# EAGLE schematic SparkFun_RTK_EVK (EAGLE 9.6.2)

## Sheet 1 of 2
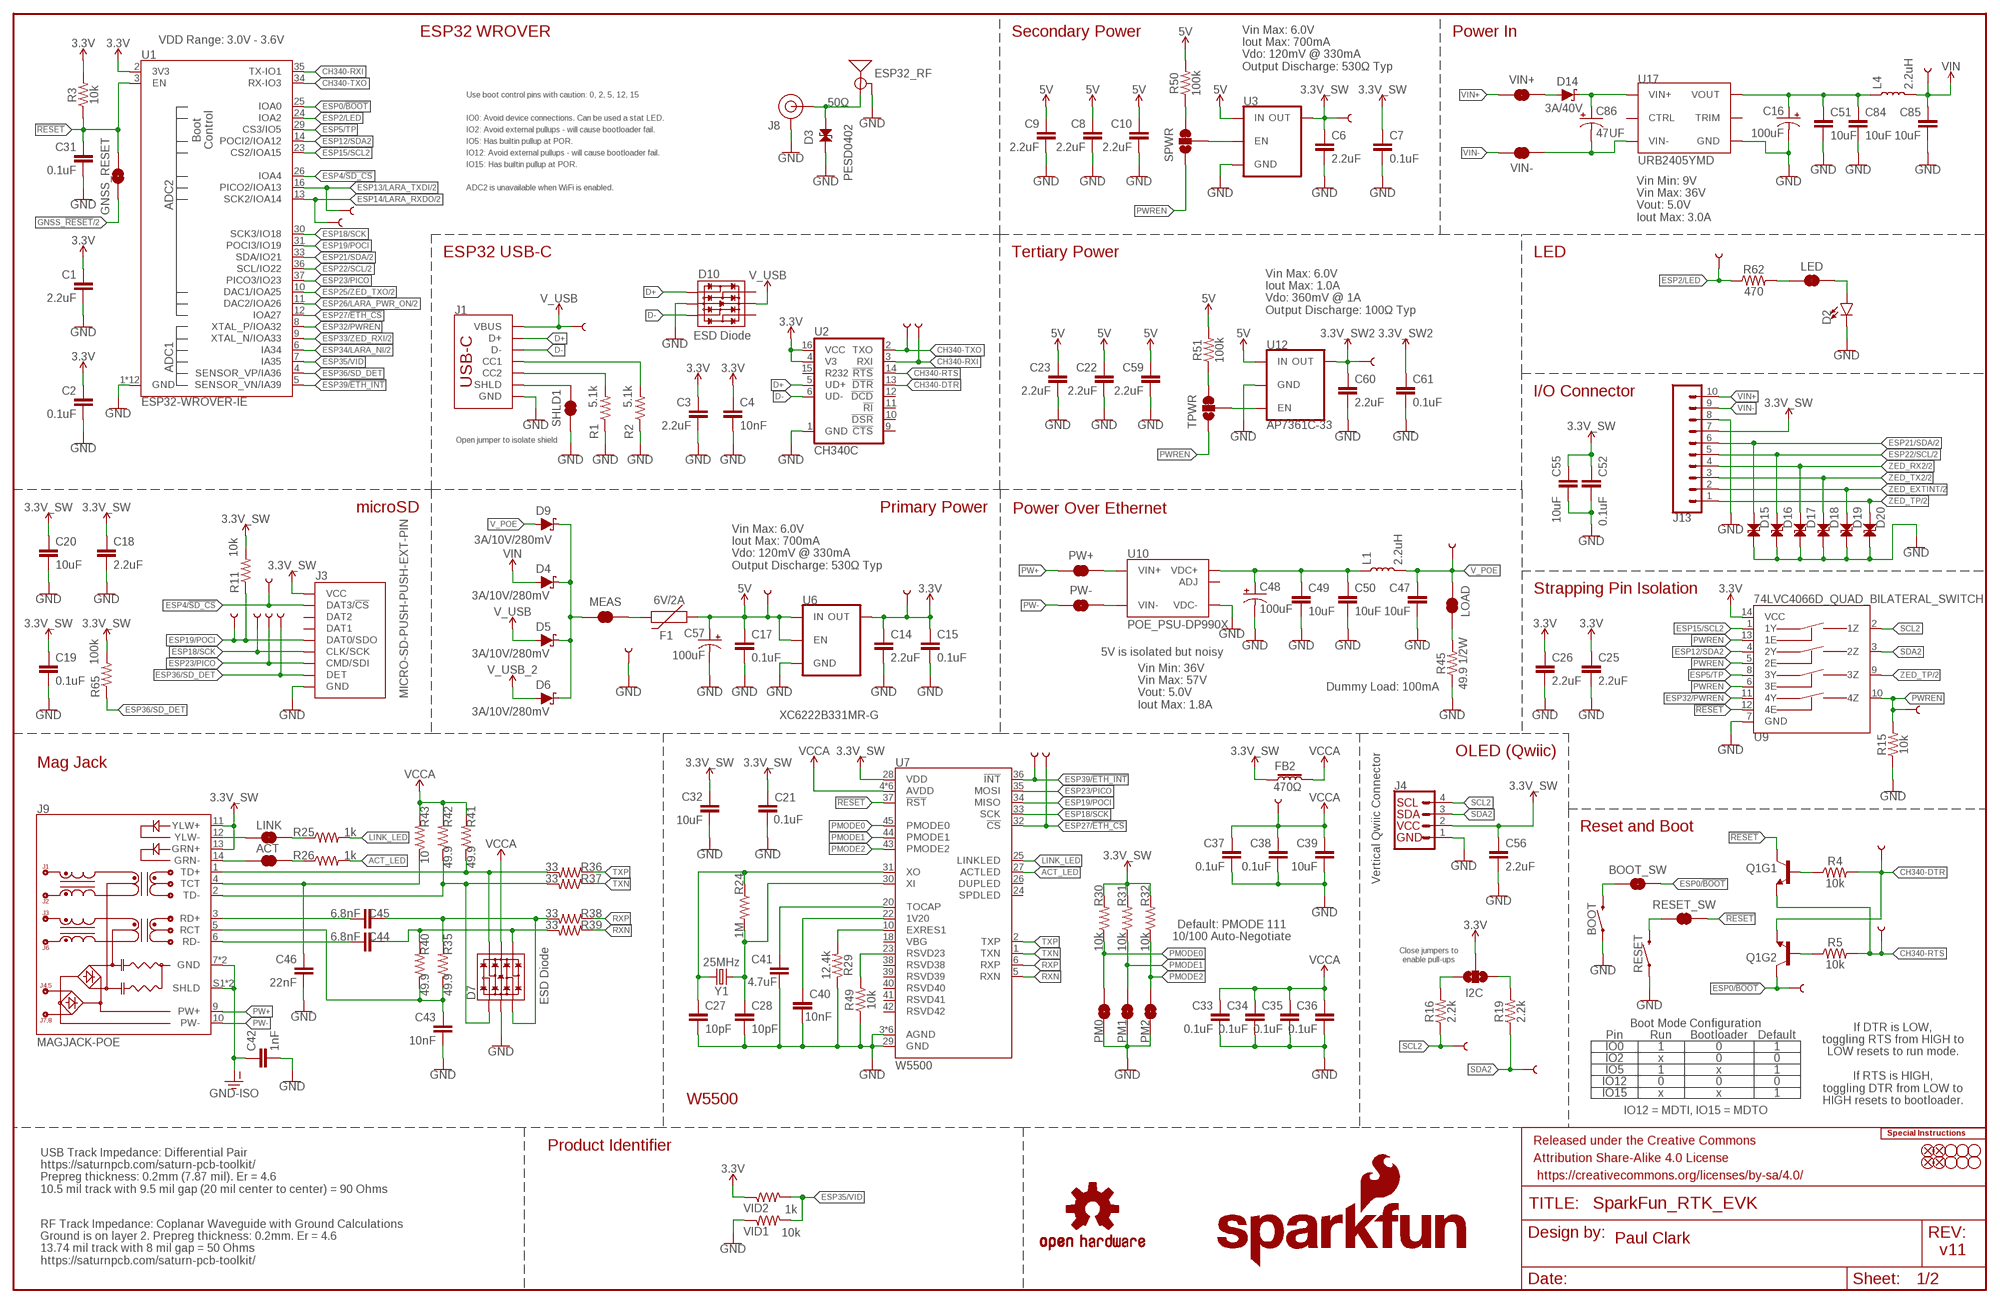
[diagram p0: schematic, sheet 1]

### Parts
3V3  TEST-POINTPOGO_PTH  [1X01_NO_SILK]
3V3_SW  TEST-POINTPOGO_PTH  [1X01_NO_SILK]
3V3_SW2  TEST-POINTPOGO_PTH  [1X01_NO_SILK]
5V  TEST-POINTPOGO_PTH  [1X01_NO_SILK]
ACT  JUMPER-SMT_2_NC_TRACE_SILK  [SMT-JUMPER_2_NC_TRACE_SILK]
BOOT  MOMENTARY-SWITCH-SPST-PTH-RIGHT-ANGLE-8-020  [TACTILE_SWITCH_PTH_RA_8-020]
BOOT_SW  JUMPER-SMT_2_NC_TRACE_SILK  [SMT-JUMPER_2_NC_TRACE_SILK]
C1  2.2uF  2.2UF-0603-10V-20%  [0603]
C2  0.1uF  0.1UF-0603-25V-5%  [0603]
C3  2.2uF  2.2UF-0603-10V-20%  [0603]
C4  10nF  10NF-0603-50V-10%  [0603]
C6  2.2uF  2.2UF-0603-10V-20%  [0603]
C7  0.1uF  0.1UF-0603-25V-5%  [0603]
C8  2.2uF  2.2UF-0603-10V-20%  [0603]
C9  2.2uF  2.2UF-0603-10V-20%  [0603]
C10  2.2uF  2.2UF-0603-10V-20%  [0603]
C14  2.2uF  2.2UF-0603-10V-20%  [0603]
C15  0.1uF  0.1UF-0603-25V-5%  [0603]
C16  100uF  100UF-POLAR-25V-20%(ELEC)  [PANASONIC_D]
C17  0.1uF  0.1UF-0603-25V-5%  [0603]
C18  2.2uF  2.2UF-0603-10V-20%  [0603]
C19  0.1uF  0.1UF-0603-25V-5%  [0603]
C20  10uF  10UF-0603-6.3V-20%  [0603]
C21  0.1uF  0.1UF-0603-25V-5%  [0603]
C22  2.2uF  2.2UF-0603-10V-20%  [0603]
C23  2.2uF  2.2UF-0603-10V-20%  [0603]
C25  2.2uF  2.2UF-0603-10V-20%  [0603]
C26  2.2uF  2.2UF-0603-10V-20%  [0603]
C27  10pF  10PF-0603-50V-5%  [0603]
C28  10pF  10PF-0603-50V-5%  [0603]
C31  0.1uF  0.1UF-0603-25V-5%  [0603]
C32  10uF  10UF-0603-6.3V-20%  [0603]
C33  0.1uF  0.1UF-0603-25V-5%  [0603]
C34  0.1uF  0.1UF-0603-25V-5%  [0603]
C35  0.1uF  0.1UF-0603-25V-5%  [0603]
C36  0.1uF  0.1UF-0603-25V-5%  [0603]
C37  0.1uF  0.1UF-0603-25V-5%  [0603]
C38  0.1uF  0.1UF-0603-25V-5%  [0603]
C39  10uF  10UF-0603-6.3V-20%  [0603]
C40  10nF  10NF-0603-50V-10%  [0603]
C41  4.7uF  4.7UF-0603-6.3V-(10%)  [0603]
C42  1nF  1.0NF/1000PF-1206-2KV-10%  [1206]
C43  10nF  10NF-0603-50V-10%  [0603]
C44  6.8nF  6.8NF/6800PF-0603-50V-5%  [0603]
C45  6.8nF  6.8NF/6800PF-0603-50V-5%  [0603]
C46  22nF  22NF/22,000PF-0603-50V-10%  [0603]
C47  10uF  10UF-0805-25V-10%  [0805]
C48  100uF  100UF-POLAR-25V-20%(ELEC)  [PANASONIC_D]
C49  10uF  10UF-0805-25V-10%  [0805]
C50  10uF  10UF-0805-25V-10%  [0805]
C51  10uF  10UF-0805-25V-10%  [0805]
C52  0.1uF  0.1UF-0603-25V-5%  [0603]
C55  10uF  10UF-0603-6.3V-20%  [0603]
C56  2.2uF  2.2UF-0603-10V-20%  [0603]
C57  100uF  100UF-POLAR-25V-20%(ELEC)  [PANASONIC_D]
C59  2.2uF  2.2UF-0603-10V-20%  [0603]
C60  2.2uF  2.2UF-0603-10V-20%  [0603]
C61  0.1uF  0.1UF-0603-25V-5%  [0603]
C84  10uF  10UF-0805-25V-10%  [0805]
C85  10uF  10UF-0805-25V-10%  [0805]
C86  47UF  47UF-POLAR-PANASONIC_D-50V-20%  [PANASONIC_D]
D2  LED-RIGHT-ANGLE-PTH-GREEN  [CBI-RIGHT-ANGLE-PTH]
D3  PESD0402  PESD0402-0402  [0402]
D4  3A/10V/280mV  DIODE-SCHOTTKY-BAT60A  [SOD-323]
D5  3A/10V/280mV  DIODE-SCHOTTKY-BAT60A  [SOD-323]
D6  3A/10V/280mV  DIODE-SCHOTTKY-BAT60A  [SOD-323]
D7  ESD Diode  TVS_DIODE_ARRAY_DT1042-04SO-7  [SOT-23-6]
D9  3A/10V/280mV  DIODE-SCHOTTKY-BAT60A  [SOD-323]
D10  ESD Diode  TVS_DIODE_ARRAY_DT1042-04SO-7  [SOT-23-6]
D14  3A/40V  DIODE-SCHOTTKY-B340A  [SMA-DIODE]
D15  PESD0402-0402  [0402]
D16  PESD0402-0402  [0402]
D17  PESD0402-0402  [0402]
D18  PESD0402-0402  [0402]
D19  PESD0402-0402  [0402]
D20  PESD0402-0402  [0402]
DET  TEST-POINTPOGO_PTH  [1X01_NO_SILK]
DTR  TEST-POINTPOGO_PTH  [1X01_NO_SILK]
ESP32_RF  ANTENNA-SMA-GROUNDEDEDGE_RPSMA  [RP-SMA-EDGE]
ETH_CS  TEST-POINTPOGO_PTH  [1X01_NO_SILK]
ETH_INT  TEST-POINTPOGO_PTH  [1X01_NO_SILK]
F1  6V/2A  PPTC_6V2A  [1210]
FB2  470Ω  FERRITE_BEAD-0603-470Ω-100MHZ-1A-200MILIΩ  [0603]
FD1  FIDUCIAL1X2  [FIDUCIAL-1X2]
FD2  FIDUCIAL1X2  [FIDUCIAL-1X2]
FD3  FIDUCIAL1X2  [FIDUCIAL-1X2]
FD4  FIDUCIAL1X2  [FIDUCIAL-1X2]
FRAME1  FRAME-LEDGER  [CREATIVE_COMMONS]
GND  TEST-POINTPOGO_PTH  [1X01_NO_SILK]
GNSS_RESET  JUMPER-COMBO_2_NO  [COMBO-JUMPER_2_NO]
H1  STAND-OFFTIGHT  [STAND-OFF-TIGHT]
H2  STAND-OFFTIGHT  [STAND-OFF-TIGHT]
H3  STAND-OFFTIGHT  [STAND-OFF-TIGHT]
H4  STAND-OFFTIGHT  [STAND-OFF-TIGHT]
H5  STAND-OFFTIGHT  [STAND-OFF-TIGHT]
H6  STAND-OFFTIGHT  [STAND-OFF-TIGHT]
I2C  JUMPER-SMT_3_NO_SILK  [SMT-JUMPER_3_NO_SILK]
J1  USB_C_4-LAYER_PADS  [USB-C-16P_4LAYER-PADS]
J3  MICRO-SD-PUSH-PUSH-EXT-PIN  [MICROSD-EXTERNALPIN]
J4  Vertical Qwiic Connector  QWIIC_CONNECTOR  [JST04_1MM_VERT]
J8  U.FL2PIN-REDUCED-FOOTPRINT  [U.FL_REDUCED_FOOTPRINT]
J9  MAGJACK-POE  [MAGJACK-SYM_LED]
J13  CONN_10_3.5MM_RA_HEADER  [1X10_SCREW_TERMINAL_3.5MM]
L1  2.2uH  INDUCTOR-0805_WIDE-2.2UH  [0805-WIDE]
L4  2.2uH  INDUCTOR-0805_WIDE-2.2UH  [0805-WIDE]
LED  JUMPER-SMT_2_NC_TRACE_SILK  [SMT-JUMPER_2_NC_TRACE_SILK]
LINK  JUMPER-SMT_2_NC_TRACE_SILK  [SMT-JUMPER_2_NC_TRACE_SILK]
LOAD  JUMPER-SMT_2_NC_TRACE_SILK  [SMT-JUMPER_2_NC_TRACE_SILK]
LOGO1  SPECIAL_INSTRUCTIONS-ORDERING  [ORDERING_INSTRUCTIONS]
LOGO4  OSHW-LOGOS  [OSHW-LOGO-S]
LOGO5  SFE_LOGO_NAME.2_INCH  [SFE_LOGO_NAME_.2]
LOGO6  SFE_LOGO_FLAME.2_INCH  [SFE_LOGO_FLAME_.2]
MEAS  JUMPER-COMBO_2_NC_TRACE  [COMBO-JUMPER_2_NC_TRACE]
PICO  TEST-POINTPOGO_PTH  [1X01_NO_SILK]
PM0  JUMPER-SMT_2_NO_SILK  [SMT-JUMPER_2_NO_SILK]
PM1  JUMPER-SMT_2_NO_SILK  [SMT-JUMPER_2_NO_SILK]
PM2  JUMPER-SMT_2_NO_SILK  [SMT-JUMPER_2_NO_SILK]
POCI  TEST-POINTPOGO_PTH  [1X01_NO_SILK]
PW+  JUMPER-COMBO_2_NC_TRACE  [COMBO-JUMPER_2_NC_TRACE]
PW-  JUMPER-COMBO_2_NC_TRACE  [COMBO-JUMPER_2_NC_TRACE]
PWREN  TEST-POINTPOGO_PTH  [1X01_NO_SILK]
Q1  TRANS_NPN_DUAL-MBT3904DW1T1  [SC70-6]
R1  5.1k  5.1KOHM5.1KOHM-0603-1/10W-1%  [0603]
R2  5.1k  5.1KOHM5.1KOHM-0603-1/10W-1%  [0603]
R3  10k  10KOHM-0603-1/10W-1%  [0603]
R4  10k  10KOHM-0603-1/10W-1%  [0603]
R5  10k  10KOHM-0603-1/10W-1%  [0603]
R11  10k  10KOHM-0603-1/10W-1%  [0603]
R15  10k  10KOHM-0603-1/10W-1%  [0603]
R16  2.2k  2.2KOHM-0603-1/10W-1%  [0603]
R19  2.2k  2.2KOHM-0603-1/10W-1%  [0603]
R24  1M  1MOHM-0603-1/4W-5%  [0603]
R25  1k  1KOHM-0603-1/10W-1%  [0603]
R26  1k  1KOHM-0603-1/10W-1%  [0603]
R29  12.4k  12.4KOHM-0603-1/10W-1%  [0603]
R30  10k  10KOHM-0603-1/10W-1%  [0603]
R31  10k  10KOHM-0603-1/10W-1%  [0603]
R32  10k  10KOHM-0603-1/10W-1%  [0603]
R35  49.9  49.9OHM-0603-1/10W-1%  [0603]
R36  33  33OHM-0603-1/10W-1%  [0603]
R37  33  33OHM-0603-1/10W-1%  [0603]
R38  33  33OHM-0603-1/10W-1%  [0603]
R39  33  33OHM-0603-1/10W-1%  [0603]
R40  49.9  49.9OHM-0603-1/10W-1%  [0603]
R41  49.9  49.9OHM-0603-1/10W-1%  [0603]
R42  49.9  49.9OHM-0603-1/10W-1%  [0603]
R43  10  10OHM-0603-1/10W-1%  [0603]
R45  49.9 1/2W  49.9OHM-1206-1/2W-1%  [1206]
R49  10k  10KOHM-0603-1/10W-1%  [0603]
R50  100k  100KOHM-0603-1/10W-1%  [0603]
R51  100k  100KOHM-0603-1/10W-1%  [0603]
R62  470  470OHM-0603-1/10W-1%  [0603]
R65  100k  100KOHM-0603-1/10W-1%  [0603]
RESET  MOMENTARY-SWITCH-SPST-PTH-RIGHT-ANGLE-8-020  [TACTILE_SWITCH_PTH_RA_8-020]
RESET_SW  JUMPER-SMT_2_NC_TRACE_SILK  [SMT-JUMPER_2_NC_TRACE_SILK]
RTS  TEST-POINTPOGO_PTH  [1X01_NO_SILK]
RX  TEST-POINTPOGO_PTH  [1X01_NO_SILK]
RXD  TEST-POINTPOGO_PTH  [1X01_NO_SILK]
SCK  TEST-POINTPOGO_PTH  [1X01_NO_SILK]
SCL2  TEST-POINTPOGO_PTH  [1X01_NO_SILK]
SD_CS  TEST-POINTPOGO_PTH  [1X01_NO_SILK]
SDA2  TEST-POINTPOGO_PTH  [1X01_NO_SILK]
SHLD1  JUMPER-SMT_2_NC_TRACE_SILK  [SMT-JUMPER_2_NC_TRACE_SILK]
SPWR  JUMPER-SMT_3_1-NC_TRACE_SILK  [SMT-JUMPER_3_1-NC_TRACE_SILK]
TP_BOOT  TEST-POINTPOGO_PTH  [1X01_NO_SILK]
TP_LED  TEST-POINTPOGO_PTH  [1X01_NO_SILK]
TPWR  JUMPER-SMT_3_1-NC_TRACE_SILK  [SMT-JUMPER_3_1-NC_TRACE_SILK]
TX  TEST-POINTPOGO_PTH  [1X01_NO_SILK]
TXD  TEST-POINTPOGO_PTH  [1X01_NO_SILK]
U1  ESP32-WROVER-IE  ESP32-WROVER-E/IE_IE-N16R8  [ESP32-WROVER-E/IE]
U2  CH340C  [SO016]
U3  XC6222B331MR-G  [SOT23-5]
U6  XC6222B331MR-G  [SOT23-5]
U7  W5500  [LQFP-48]
U9  74LVC4066D_QUAD_BILATERAL_SWITCH  [SO14]
U10  POE_PSU-DP990X  [DP990X]
U12  AP7361C-33  AP7361C-33FGEUDFN-8  [UDFN-8]
U17  URB2405YMD  URB_YMD-15WR3__URB2405YMD-15WR3  [URB_YMD-15WR3]
VCCA  TEST-POINTPOGO_PTH  [1X01_NO_SILK]
VID1  10k  10KOHM-0603-1/10W-1%  [0603]
VID2  1k  1KOHM-0603-1/10W-1%  [0603]
VIN  TEST-POINTPOGO_PTH  [1X01_NO_SILK]
VIN+  JUMPER-COMBO_2_NC_TRACE  [COMBO-JUMPER_2_NC_TRACE]
VIN-  JUMPER-COMBO_2_NC_TRACE  [COMBO-JUMPER_2_NC_TRACE]
VPOE  TEST-POINTPOGO_PTH  [1X01_NO_SILK]
VUSB  TEST-POINTPOGO_PTH  [1X01_NO_SILK]
Y1  25MHz  CRYSTAL-25MHZ-SMD-2.0X1.6MM  [CRYSTAL-SMD-2.0X1.6MM]

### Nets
3.3V: 3V3.1 C1.1 C2.1 C3.1 C4.1 C14.1 C15.1 C25.1 C26.1 I2C.2 R3.2 U1.2(3V3) U2.4(V3) U2.16(VCC) U6.5(OUT) U9.14(VCC) VID2.1
3.3V_SW: 3V3_SW.1 C6.1 C7.1 C18.1 C19.1 C20.1 C21.1 C32.1 C52.1 C55.1 C56.1 FB2.1 J3.4(VCC) J4.2 J9.11(YLW+) J9.13(GRN+) J13.7 R11.2 R30.2 R31.2 R32.2 R65.2 U3.5(OUT) U7.28(VDD) ; also sheet 2
3.3V_SW2: 3V3_SW2.1 C60.1 C61.1 U12.1(OUT) ; also sheet 2
5V: 5V.1 C8.1 C9.1 C10.1 C17.1 C22.1 C23.1 C57.+ C59.1 F1.1 R50.2 R51.2 U3.1(IN) U6.1(IN) U6.3(EN) U12.8(IN) ; also sheet 2
5V_RAW: C48.+ C49.1 C50.1 L1.1 U10.1(VDC+) U10.2(VDC+)
5V_RAW1: C16.+ C51.1 C84.1 L4.1 U17.4(VOUT)
!RESET!: C31.1 GNSS_RESET.2 GNSS_RESET.4 Q1.3(C) R3.1 RESET_SW.1 U1.3(EN) U7.37(!RST!) U9.12(4E)
ACT: ACT.1 J9.14(GRN-)
ACT_LED: R26.2 U7.27(ACTLED)
CH340-DTR: DTR.1 Q1.1(E) R4.2 U2.13(!DTR)
CH340-RTS: Q1.4(E) R5.2 RTS.1 U2.14(!RTS)
CH340-RXI: TX.1 U1.35(TX-IO1) U2.3(RXI)
CH340-TXO: RX.1 U1.34(RX-IO3) U2.2(TXO)
D+: D10.1(IO1) J1.A6(D+) J1.B6(D+) U2.5(UD+)
D-: D10.3(IO2) J1.A7(D-) J1.B7(D-) U2.6(UD-)
ESP0/!BOOT!: BOOT_SW.1 Q1.6(C) TP_BOOT.1 U1.25(IOA0)
ESP2/LED: R62.1 TP_LED.1 U1.24(IOA2)
ESP4/!SD_CS!: J3.2(DAT3/!CS!) SD_CS.1 U1.26(IOA4)
ESP5/TP: U1.29(CS3/IO5) U9.8(3Y)
ESP12/SDA2: U1.14(POCI2/IOA12) U9.4(2Y)
ESP13/LARA_TXDI: TXD.1 U1.16(PICO2/IOA13) ; also sheet 2
ESP14/LARA_RXDO: RXD.1 U1.13(SCK2/IOA14) ; also sheet 2
ESP15/SCL2: U1.23(CS2/IOA15) U9.1(1Y)
ESP18/SCK: J3.5(CLK/SCK) SCK.1 U1.30(SCK3/IO18) U7.33(SCK)
ESP19/POCI: J3.7(DAT0/SDO) POCI.1 R11.1 U1.31(POCI3/IO19) U7.34(MISO)
ESP21/SDA: D15.1 J13.6 U1.33(SDA/IO21) ; also sheet 2
ESP22/SCL: D16.1 J13.5 U1.36(SCL/IO22) ; also sheet 2
ESP23/PICO: J3.3(CMD/SDI) PICO.1 U1.37(PICO3/IO23) U7.35(MOSI)
ESP25/ZED_TXO: U1.10(DAC1/IOA25) ; also sheet 2
ESP26/LARA_PWR_ON: U1.11(DAC2/IOA26) ; also sheet 2
ESP27/!ETH_CS!: ETH_CS.1 U1.12(IOA27) U7.32(!CS!)
ESP32/PWREN: U1.8(XTAL_P/IOA32) U9.11(4Y)
ESP33/ZED_RXI: U1.9(XTAL_N/IOA33) ; also sheet 2
ESP34/LARA_NI: U1.6(IA34) ; also sheet 2
ESP35/VID: U1.7(IA35) VID1.2 VID2.2
ESP36/SD_DET: DET.1 J3.9(DET) R65.1 U1.4(SENSOR_VP/IA36)
ESP39/!ETH_INT!: ETH_INT.1 U1.5(SENSOR_VN/IA39) U7.36(!INT!)
GND: BOOT.1 C1.2 C2.2 C3.2 C4.2 C6.2 C7.2 C8.2 C9.2 C10.2 C14.2 C15.2 C16.- C17.2 C18.2 C19.2 C20.2 C21.2 C22.2 C23.2 C25.2 C26.2 C27.2 C28.2 C31.2 C32.2 C33.2 C34.2 C35.2 C36.2 C37.2 C38.2 C39.2 C40.2 C41.2 C42.2 C43.2 C46.2 C47.2 C48.- C49.2 C50.2 C51.2 C52.2 C55.2 C56.2 C57.- C59.2 C60.2 C61.2 C84.2 C85.2 D2.C D3.2 D7.2(VSS) D10.2(VSS) D15.2 D16.2 D17.2 D18.2 D19.2 D20.2 ESP32_RF.GND@0(GND) ESP32_RF.GND@1(GND) ESP32_RF.GND@2(GND) ESP32_RF.GND@3(GND) GND.1 J1.GND J1.GND2(GND) J3.6(GND) J3.10(GND) J3.11(GND) J3.12(GND) J3.13(GND) J4.1 J8.1(GND) J8.2(GND) J13.8 PM0.1 PM1.1 PM2.1 R1.1 R2.1 R15.1 R29.1 R45.1 R49.1 RESET.1 SHLD1.1 U1.1(GND) U1.15(GND) U1.38(GND) U1.GND U1.GNDT1(GND) U1.GNDT2(GND) U1.GNDT3(GND) U1.GNDT4(GND) U1.GNDT5(GND) U1.GNDT6(GND) U1.GNDT7(GND) U1.GNDT8(GND) U2.1(GND) U3.2(GND) U6.2(GND) U7.3(AGND) U7.9(AGND) U7.14(AGND) U7.16(AGND) U7.19(AGND) U7.29(GND) U7.48(AGND) U9.7(GND) U10.3(VDC-) U12.4(GND) U12.EP(GND) U17.6(GND) VID1.1 ; also sheet 2
GND-ISO: C42.1 J9.7(GND) J9.8(GND) J9.S1(SHLD) J9.S2(SHLD)
GNSS_!RESET!: GNSS_RESET.1 GNSS_RESET.3 ; also sheet 2
LINK: J9.12(YLW-) LINK.1
LINK_LED: R25.2 U7.25(LINKLED)
MEAS: D4.C D5.C D6.C D9.C MEAS.2 MEAS.4
N$1: J1.B5(CC2) R1.2
N$2: J1.A5(CC1) R2.2
N$4: Q1.2(B) R5.1
N$5: Q1.5(B) R4.1
N$7: LED.2 R62.2
N$10: F1.2 MEAS.1 MEAS.3
N$12: ACT.2 R26.1
N$13: D3.1 ESP32_RF.SIG(SIGNAL) J8.FEED(SIGNAL)
N$14: I2C.3 R16.2
N$15: I2C.1 R19.2
N$19: C27.1 R24.1 U7.31(XO) Y1.1
N$20: C28.1 R24.2 U7.30(XI) Y1.3
N$21: LINK.2 R25.1
N$22: R50.1 SPWR.3
N$23: R29.2 U7.10(EXRES1)
N$24: C40.1 U7.22(1V20)
N$25: C41.1 U7.20(TOCAP)
N$26: SPWR.2 U3.3(EN)
N$27: LOAD.1 R45.2
N$28: RESET.2 RESET_SW.2
N$29: BOOT.2 BOOT_SW.2
N$30: R49.2 U7.23(RSVD23)
N$31: R51.1 TPWR.3
N$39: TPWR.2 U12.5(EN)
N$45: D2.A LED.1
PMODE0: PM0.2 R30.1 U7.45(PMODE0)
PMODE1: PM1.2 R31.1 U7.44(PMODE1)
PMODE2: PM2.2 R32.1 U7.43(PMODE2)
PW1+: PW+.1 PW+.3 U10.5(VIN+) U10.6(VIN+)
PW1-: PW-.1 PW-.3 U10.7(VIN-) U10.8(VIN-)
PW+: J9.9(PW+) PW+.2 PW+.4
PW-: J9.10(PW-) PW-.2 PW-.4
PWREN: PWREN.1 R15.2 SPWR.1 TPWR.1 U9.5(2E) U9.6(3E) U9.10(4Z) U9.13(1E)
RCT: C43.1 J9.5(RCT) R35.1 R40.1
RD+: C45.2 J9.3(RD+)
RD-: C44.2 J9.6(RD-)
RXN: R39.1 U7.5(RXN)
RXN1: C44.1 D7.4(IO3) R39.2 R40.2
RXP: R38.1 U7.6(RXP)
RXP1: C45.1 D7.3(IO2) R35.2 R38.2
SCL2: J4.4 R16.1 SCL2.1 U9.2(1Z)
SDA2: J4.3 R19.1 SDA2.1 U9.3(2Z)
SHIELD: J1.SHLD1(SHLD) J1.SHLD2(SHLD) J1.SHLD3(SHLD) J1.SHLD4(SHLD) SHLD1.2
TCT: C46.1 J9.4(TCT) R43.1
TD+: D7.6(IO4) J9.1(TD+) R36.2 R41.1
TD-: D7.1(IO1) J9.2(TD-) R37.2 R42.1
TXN: R37.1 U7.1(TXN)
TXP: R36.1 U7.2(TXP)
V_POE: C47.1 D9.A L1.2 LOAD.2 VPOE.1
V_USB: D5.A D10.5(VCC) J1.VBUS1(VBUS) J1.VBUS2(VBUS) VUSB.1
V_USB_2: D6.A ; also sheet 2
VCCA: C33.1 C34.1 C35.1 C36.1 C37.1 C38.1 C39.1 D7.5(VCC) FB2.2 R41.2 R42.2 R43.2 U7.4(AVDD) U7.8(AVDD) U7.11(AVDD) U7.15(AVDD) U7.17(AVDD) U7.21(AVDD) VCCA.1
VIN: C85.1 D4.A L4.2 VIN.1
VIN1+: D14.A VIN+.1 VIN+.3
VIN1-: C86.- U17.2(VIN-) VIN-.2 VIN-.4
VIN2+: C86.+ D14.C U17.3(VIN+)
VIN+: J13.10 VIN+.2 VIN+.4
VIN-: J13.9 VIN-.1 VIN-.3
ZED_EXTINT: D19.1 J13.2 ; also sheet 2
ZED_RX2: D17.1 J13.4 ; also sheet 2
ZED_TP: D20.1 J13.1 U9.9(3Z) ; also sheet 2
ZED_TX2: D18.1 J13.3 ; also sheet 2
Unconnected: D10.4(IO3) D10.6(IO4) J3.1(DAT2) J3.8(DAT1) U2.9(!CTS) U2.10(!DSR) U2.11(!RI) U2.12(!DCD) U2.15(R232) U7.18(VBG) U7.24(SPDLED) U7.26(DUPLED) U7.38(RSVD38) U7.39(RSVD39) U7.40(RSVD40) U7.41(RSVD41) U7.42(RSVD42) U10.4(ADJ) U17.1(CTRL) U17.5(TRIM)

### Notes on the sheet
- Secondary Power | Power In
- VDD Range: 3.0V - 3.6V | ESP32 WROVER
- Vin Max: 6.0V
  Iout Max: 700mA
  Vdo: 120mV @ 330mA
  Output Discharge: 530Ω Typ
- Use boot control pins with caution: 0, 2, 5, 12, 15
- 50Ω
- IO0: Avoid device connections. Can be used a stat LED.
- IO2: Avoid external pullups - will cause bootloader fail.
- IO5: Has builtin pullup at POR.
- IO12: Avoid external pullups - will cause bootloader fail.
- IO15: Has builtin pullup at POR.
- ADC2 is unavailable when WiFi is enabled.
- Vin Min: 9V
  Vin Max: 36V
  Vout: 5.0V
  Iout Max: 3.0A
- ESP32 USB-C | Tertiary Power | LED
- Vin Max: 6.0V
  Iout Max: 1.0A
  Vdo: 360mV @ 1A
  Output Discharge: 100Ω Typ
- I/O Connector
- Open jumper to isolate shield
- microSD | Primary Power | Power Over Ethernet
- Vin Max: 6.0V
  Iout Max: 700mA
  Vdo: 120mV @ 330mA
  Output Discharge: 530Ω Typ
- Strapping Pin Isolation
- 5V is isolated but noisy
- Dummy Load: 100mA
- Vin Min: 36V
  Vin Max: 57V
  Vout: 5.0V
  Iout Max: 1.8A
- OLED (Qwiic)
- Mag Jack
- Reset and Boot
- Default: PMODE 111
  10/100 Auto-Negotiate
- Close jumpers to
  enable pull-ups
- Boot Mode Configuration
- If DTR is LOW,
  toggling RTS from HIGH to
  LOW resets to run mode.
  
  If RTS is HIGH,
  toggling DTR from LOW to
  HIGH resets to bootloader.
- Pin | Run | Bootloader | Default
- IO0 | 1 | 0 | 1
- IO2 | x | 0 | 0
- IO5 | 1 | x | 1
- IO12 | 0 | 0 | 0
- IO15 | x | x | 1
- W5500
- IO12 = MDTI, IO15 = MDTO
- Product Identifier
- USB Track Impedance: Differential Pair
  https://saturnpcb.com/saturn-pcb-toolkit/
  Prepreg thickness: 0.2mm (7.87 mil). Er = 4.6
  10.5 mil track with 9.5 mil gap (20 mil center to center) = 90 Ohms
- Paul Clark
- v11
- RF Track Impedance: Coplanar Waveguide with Ground Calculations
  Ground is on layer 2. Prepreg thickness: 0.2mm. Er = 4.6
  13.74 mil track with 8 mil gap = 50 Ohms
  https://saturnpcb.com/saturn-pcb-toolkit/

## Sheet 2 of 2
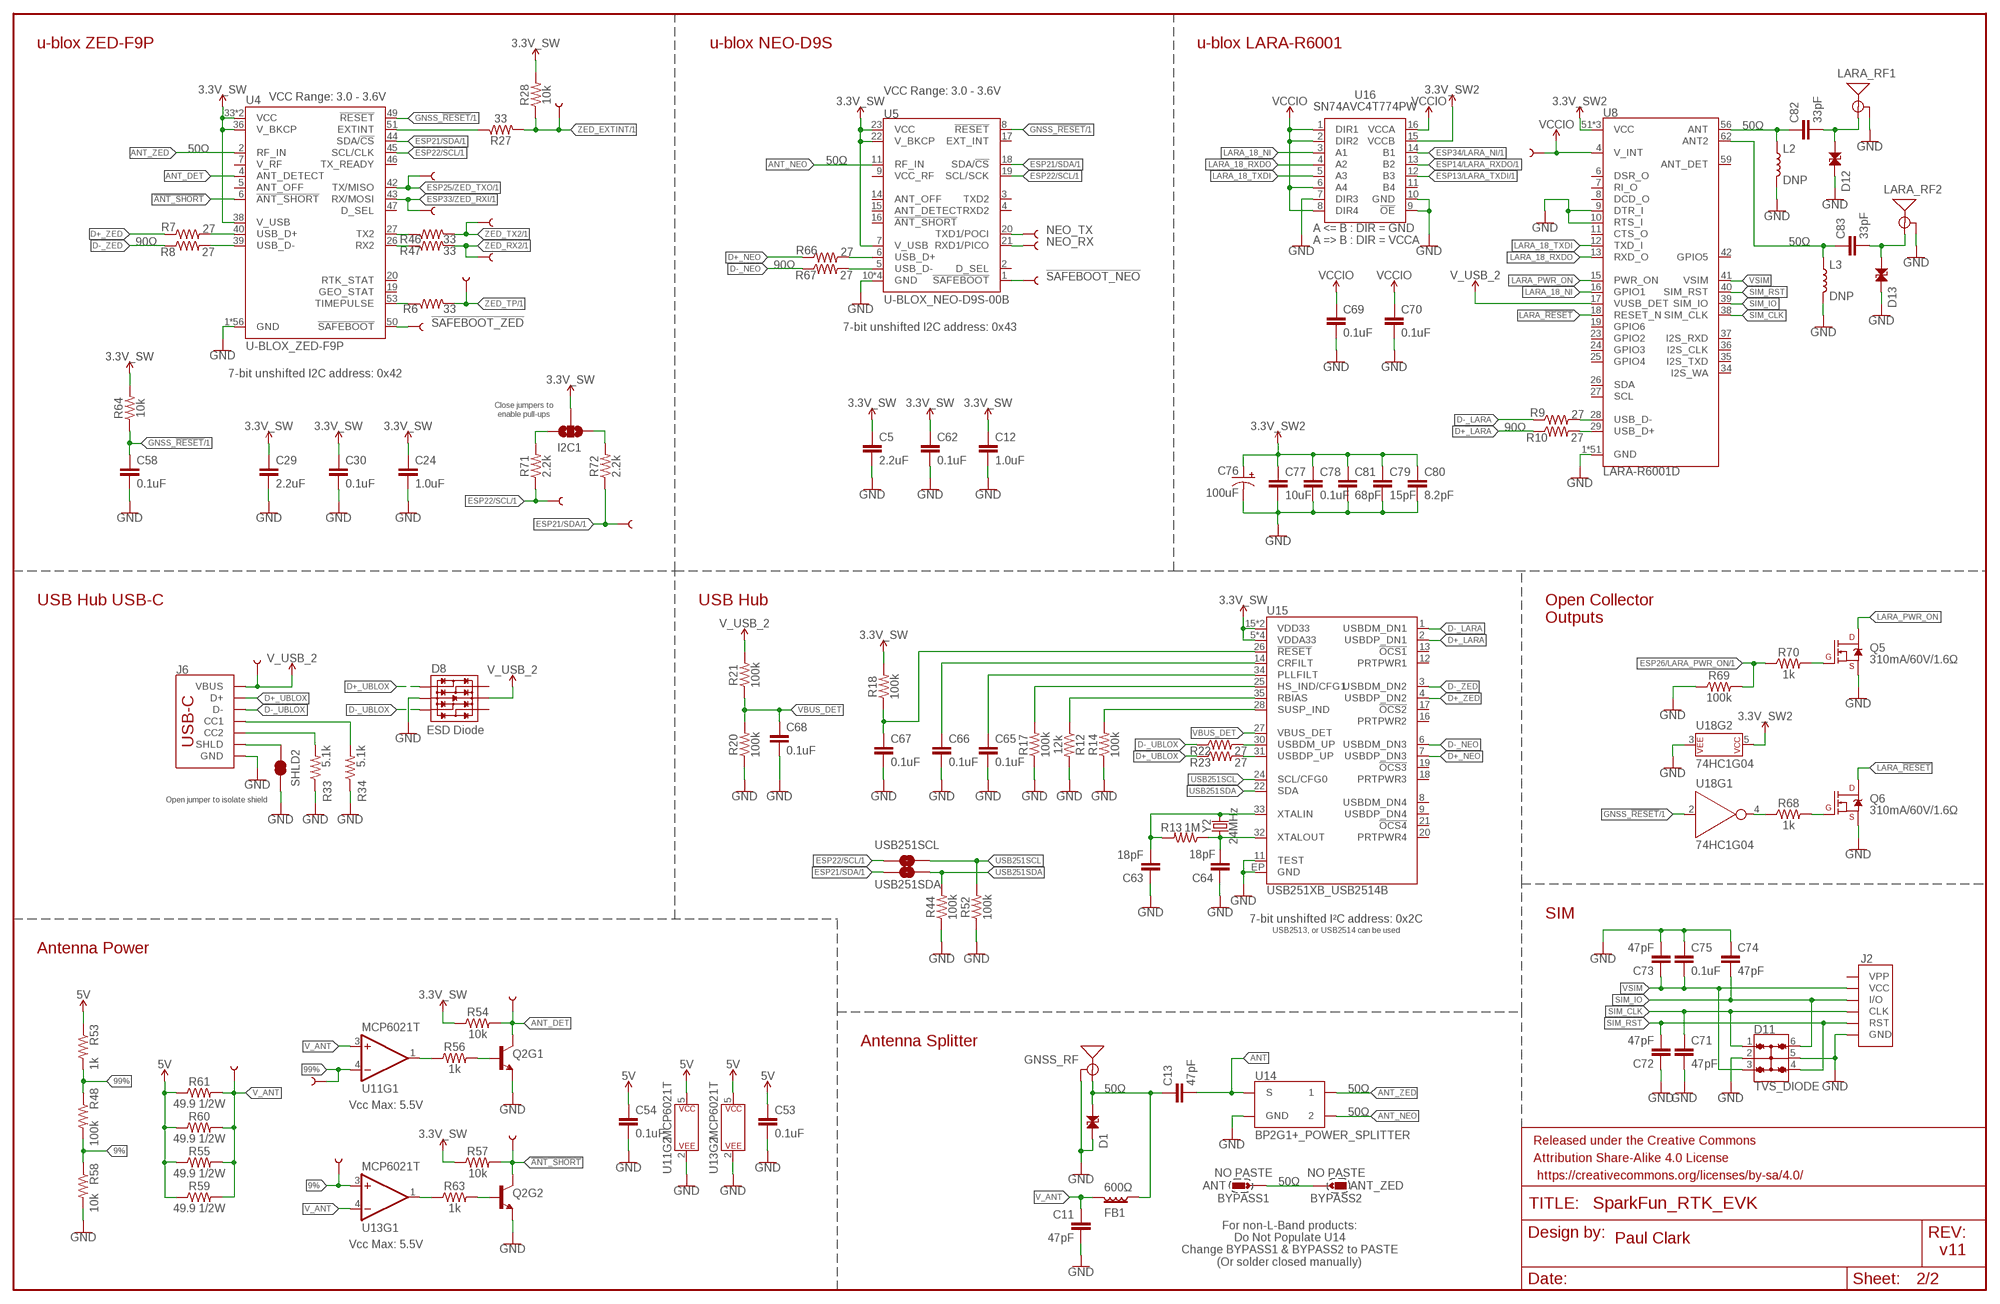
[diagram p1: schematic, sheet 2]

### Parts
9%  TEST-POINTPOGO_PTH  [1X01_NO_SILK]
99%  TEST-POINTPOGO_PTH  [1X01_NO_SILK]
!SAFEBOOT_NEO!  TEST-POINTPOGO_PTH  [1X01_NO_SILK]
!SAFEBOOT_ZED!  TEST-POINTPOGO_PTH  [1X01_NO_SILK]
ANT_DET  TEST-POINTPOGO_PTH  [1X01_NO_SILK]
ANT_SHT  TEST-POINTPOGO_PTH  [1X01_NO_SILK]
BYPASS1  NO PASTE  JUMPER-SMT_2_SOIC-PAD_NO-PASTE  [SMT-JUMPER_2_SOIC-PAD_NO-PASTE]
BYPASS2  NO PASTE  JUMPER-SMT_2_SOIC-PAD_NO-PASTE  [SMT-JUMPER_2_SOIC-PAD_NO-PASTE]
C5  2.2uF  2.2UF-0603-10V-20%  [0603]
C11  47pF  47PF-0603-50V-5%  [0603]
C12  1.0uF  1.0UF-0603-16V-10%  [0603]
C13  47pF  47PF-0603-50V-5%  [0603]
C24  1.0uF  1.0UF-0603-16V-10%  [0603]
C29  2.2uF  2.2UF-0603-10V-20%  [0603]
C30  0.1uF  0.1UF-0603-25V-5%  [0603]
C53  0.1uF  0.1UF-0603-25V-5%  [0603]
C54  0.1uF  0.1UF-0603-25V-5%  [0603]
C58  0.1uF  0.1UF-0603-25V-5%  [0603]
C62  0.1uF  0.1UF-0603-25V-5%  [0603]
C63  18pF  18PF-0603-50V-5%  [0603]
C64  18pF  18PF-0603-50V-5%  [0603]
C65  0.1uF  0.1UF-0603-25V-5%  [0603]
C66  0.1uF  0.1UF-0603-25V-5%  [0603]
C67  0.1uF  0.1UF-0603-25V-5%  [0603]
C68  0.1uF  0.1UF-0603-25V-5%  [0603]
C69  0.1uF  0.1UF-0603-25V-5%  [0603]
C70  0.1uF  0.1UF-0603-25V-5%  [0603]
C71  47pF  47PF-0603-50V-5%  [0603]
C72  47pF  47PF-0603-50V-5%  [0603]
C73  47pF  47PF-0603-50V-5%  [0603]
C74  47pF  47PF-0603-50V-5%  [0603]
C75  0.1uF  0.1UF-0603-25V-5%  [0603]
C76  100uF  100UF-POLAR-25V-20%(ELEC)  [PANASONIC_D]
C77  10uF  10UF-0805-25V-10%  [0805]
C78  0.1uF  0.1UF-0603-25V-5%  [0603]
C79  15pF  15PF-0603-50V-5%  [0603]
C80  8.2pF  8.2PF-0603-50V-10%  [0603]
C81  68pF  68PF-0603-50V-5%  [0603]
C82  33pF  33PF-0603-50V-5%  [0603]
C83  33pF  33PF-0603-50V-5%  [0603]
D1  PESD0402-0402  [0402]
D8  ESD Diode  TVS_DIODE_ARRAY_DT1042-04SO-7  [SOT-23-6]
D11  TVS_DIODE  TVS_DIODE_ARRAY_4_ESDA6V1BC6  [SOT23-6L]
D12  PESD0402-0402  [0402]
D13  PESD0402-0402  [0402]
FB1  600Ω  FERRITE_BEAD-0805-600Ω-100MHZ  [0805]
FRAME2  FRAME-LEDGERNO_FOOTPRINT  [DUMMY]
GNSS_RF  ANTENNA-SMA-GROUNDEDEDGE_SMA  [SMA-EDGE]
I2C1  JUMPER-SMT_3_NO_SILK  [SMT-JUMPER_3_NO_SILK]
J2  SIMHOLDER-PUSHPUSH  [NANO_SIM_PP]
J6  USB_C_4-LAYER_PADS  [USB-C-16P_4LAYER-PADS]
L2  DNP  DNP-0603_NO-CREAM  [0603_NO-CREAM]
L3  DNP  DNP-0603_NO-CREAM  [0603_NO-CREAM]
LARA_RF1  ANTENNA-SMA-GROUNDEDEDGE_SMA  [SMA-EDGE]
LARA_RF2  ANTENNA-SMA-GROUNDEDEDGE_SMA  [SMA-EDGE]
NEO_RX  TEST-POINTPOGO_PTH  [1X01_NO_SILK]
NEO_TX  TEST-POINTPOGO_PTH  [1X01_NO_SILK]
Q2  TRANS_NPN_DUAL-MBT3904DW1T1  [SC70-6]
Q5  310mA/60V/1.6Ω  MOSFET-NCH-2N7002PW  [SOT323]
Q6  310mA/60V/1.6Ω  MOSFET-NCH-2N7002PW  [SOT323]
R6  33  33OHM-0603-1/10W-1%  [0603]
R7  27  27OHM-0603-1/10W-1%  [0603]
R8  27  27OHM-0603-1/10W-1%  [0603]
R9  27  27OHM-0603-1/10W-1%  [0603]
R10  27  27OHM-0603-1/10W-1%  [0603]
R12  12k  12KOHM-0603-1/10W-1%  [0603]
R13  1M  1MOHM-0603-1/4W-5%  [0603]
R14  100k  100KOHM-0603-1/10W-1%  [0603]
R17  100k  100KOHM-0603-1/10W-1%  [0603]
R18  100k  100KOHM-0603-1/10W-1%  [0603]
R20  100k  100KOHM-0603-1/10W-1%  [0603]
R21  100k  100KOHM-0603-1/10W-1%  [0603]
R22  27  27OHM-0603-1/10W-1%  [0603]
R23  27  27OHM-0603-1/10W-1%  [0603]
R27  33  33OHM-0603-1/10W-1%  [0603]
R28  10k  10KOHM-0603-1/10W-1%  [0603]
R33  5.1k  5.1KOHM5.1KOHM-0603-1/10W-1%  [0603]
R34  5.1k  5.1KOHM5.1KOHM-0603-1/10W-1%  [0603]
R44  100k  100KOHM-0603-1/10W-1%  [0603]
R46  33  33OHM-0603-1/10W-1%  [0603]
R47  33  33OHM-0603-1/10W-1%  [0603]
R48  100k  100KOHM-0603-1/10W-1%  [0603]
R52  100k  100KOHM-0603-1/10W-1%  [0603]
R53  1k  1KOHM-0603-1/10W-1%  [0603]
R54  10k  10KOHM-0603-1/10W-1%  [0603]
R55  49.9 1/2W  49.9OHM-1206-1/2W-1%  [1206]
R56  1k  1KOHM-0603-1/10W-1%  [0603]
R57  10k  10KOHM-0603-1/10W-1%  [0603]
R58  10k  10KOHM-0603-1/10W-1%  [0603]
R59  49.9 1/2W  49.9OHM-1206-1/2W-1%  [1206]
R60  49.9 1/2W  49.9OHM-1206-1/2W-1%  [1206]
R61  49.9 1/2W  49.9OHM-1206-1/2W-1%  [1206]
R63  1k  1KOHM-0603-1/10W-1%  [0603]
R64  10k  10KOHM-0603-1/10W-1%  [0603]
R66  27  27OHM-0603-1/10W-1%  [0603]
R67  27  27OHM-0603-1/10W-1%  [0603]
R68  1k  1KOHM-0603-1/10W-1%  [0603]
R69  100k  100KOHM-0603-1/10W-1%  [0603]
R70  1k  1KOHM-0603-1/10W-1%  [0603]
R71  2.2k  2.2KOHM-0603-1/10W-1%  [0603]
R72  2.2k  2.2KOHM-0603-1/10W-1%  [0603]
RX2  TEST-POINTPOGO_PTH  [1X01_NO_SILK]
SCL  TEST-POINTPOGO_PTH  [1X01_NO_SILK]
SDA  TEST-POINTPOGO_PTH  [1X01_NO_SILK]
SHLD2  JUMPER-SMT_2_NC_TRACE_SILK  [SMT-JUMPER_2_NC_TRACE_SILK]
TP  TEST-POINTPOGO_PTH  [1X01_NO_SILK]
TX2  TEST-POINTPOGO_PTH  [1X01_NO_SILK]
U4  U-BLOX_ZED-F9P  [ZED-F9P]
U5  U-BLOX_NEO-D9S-00B  [NEO-M9N/M8T/M8U/D9S]
U8  LARA-R6001D  LARA-R6_R6001D_GLOBAL_DATA-ONLY  [LARA-LGA]
U11  MCP6021T  MCP6021T-E/OT  [SOT23-5]
U13  MCP6021T  MCP6021T-E/OT  [SOT23-5]
U14  BP2G1+_POWER_SPLITTER  [XX21]
U15  USB251XB_USB2514B  [QFN-36]
U16  SN74AVC4T774PW  [SOP65P640X120-16N]
U18  74HC1G04  [SOT353]
USB251SCL  JUMPER-SMT_2_NO_SILK  [SMT-JUMPER_2_NO_SILK]
USB251SDA  JUMPER-SMT_2_NO_SILK  [SMT-JUMPER_2_NO_SILK]
VANT  TEST-POINTPOGO_PTH  [1X01_NO_SILK]
VCCIO  TEST-POINTPOGO_PTH  [1X01_NO_SILK]
VUSB2  TEST-POINTPOGO_PTH  [1X01_NO_SILK]
Y2  24MHz  CRYSTAL-24MHZ-SMD-2.0X1.6MM  [CRYSTAL-SMD-2.0X1.6MM]
ZED_EXTINT  TEST-POINTPOGO_PTH  [1X01_NO_SILK]
ZED_RXI  TEST-POINTPOGO_PTH  [1X01_NO_SILK]
ZED_TXO  TEST-POINTPOGO_PTH  [1X01_NO_SILK]

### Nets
3.3V_SW: C5.1 C12.1 C24.1 C29.1 C30.1 C62.1 I2C1.2 R18.2 R28.2 R54.1 R57.1 R64.2 U4.33(VCC) U4.34(VCC) U4.36(V_BKCP) U4.38(V_USB) U5.7(V_USB) U5.22(V_BKCP) U5.23(VCC) U15.5(VDDA33) U15.10(VDDA33) U15.15(VDD33) U15.23(VDD33) U15.29(VDDA33) U15.36(VDDA33) ; also sheet 1
3.3V_SW2: C76.+ C77.1 C78.1 C79.1 C80.1 C81.1 U8.51(VCC) U8.52(VCC) U8.53(VCC) U16.15(VCCB) U18.5(P$V+) ; also sheet 1
5V: C53.1 C54.1 R53.1 R55.1 R59.1 R60.1 R61.1 U11.5(P$V+) U13.5(P$V+) ; also sheet 1
9%: 9%.1 R48.2 R58.1 U13.3(+IN)
99%: 99%.1 R48.1 R53.2 U11.4(-IN)
!ANT_SHORT!: ANT_SHT.1 Q2.6(C) R57.2 U4.6(!ANT_SHORT!)
!SAFEBOOT_NEO!: !SAFEBOOT_NEO!.1 U5.1(!SAFEBOOT!)
!SAFEBOOT_ZED!: !SAFEBOOT_ZED!.1 U4.50(!SAFEBOOT!)
ANT: C13.2 U14.2(S)
ANT_DET: ANT_DET.1 Q2.3(C) R54.2 U4.4(ANT_DETECT)
ANT_NEO: U5.11(RF_IN) U14.5
ANT_ZED: U4.2(RF_IN) U14.8
BYPASS: BYPASS1.1 BYPASS2.1
D+_LARA: R10.1 U15.2(USBDP_DN1)
D+_NEO: R66.1 U15.7(USBDP_DN3)
D+_UBLOX: D8.1(IO1) J6.A6(D+) J6.B6(D+) R23.1
D+_ZED: R7.1 U15.4(USBDP_DN2)
D-_LARA: R9.1 U15.1(USBDM_DN1)
D-_NEO: R67.1 U15.6(USBDM_DN3)
D-_UBLOX: D8.3(IO2) J6.A7(D-) J6.B7(D-) R22.1
D-_ZED: R8.1 U15.3(USBDM_DN2)
ESP13/LARA_TXDI: U16.12(B3) ; also sheet 1
ESP14/LARA_RXDO: U16.13(B2) ; also sheet 1
ESP21/SDA: R72.1 SDA.1 U4.44(SDA/!CS!) U5.18(SDA/!CS!) USB251SDA.1 ; also sheet 1
ESP22/SCL: R71.1 SCL.1 U4.45(SCL/CLK) U5.19(SCL/SCK) USB251SCL.1 ; also sheet 1
ESP25/ZED_TXO: U4.42(TX/MISO) ZED_TXO.1 ; also sheet 1
ESP26/LARA_PWR_ON: R69.2 R70.1 ; also sheet 1
ESP33/ZED_RXI: U4.43(RX/MOSI) ZED_RXI.1 ; also sheet 1
ESP34/LARA_NI: U16.14(B1) ; also sheet 1
GND: C5.2 C11.2 C12.2 C24.2 C29.2 C30.2 C53.2 C54.2 C58.2 C62.2 C63.1 C64.1 C65.2 C66.2 C67.2 C68.2 C69.2 C70.2 C71.2 C72.1 C73.2 C74.1 C75.1 C76.- C77.2 C78.2 C79.2 C80.2 C81.2 D1.2 D8.2(VSS) D11.2 D11.5 D12.2 D13.2 GNSS_RF.GND@0(GND) GNSS_RF.GND@1(GND) GNSS_RF.GND@2(GND) GNSS_RF.GND@3(GND) J2.C5(GND) J6.GND J6.GND2(GND) L2.2 L3.2 LARA_RF1.GND@0(GND) LARA_RF1.GND@1(GND) LARA_RF1.GND@2(GND) LARA_RF1.GND@3(GND) LARA_RF2.GND@0(GND) LARA_RF2.GND@1(GND) LARA_RF2.GND@2(GND) LARA_RF2.GND@3(GND) Q2.1(E) Q2.4(E) Q5.2(S) Q6.2(S) R12.2 R14.1 R17.1 R20.1 R33.1 R34.1 R44.1 R52.1 R58.2 R69.1 SHLD2.1 U4.1(GND) U4.3(GND) U4.12(GND) U4.14(GND) U4.32(GND) U4.37(GND) U4.41(GND) U4.48(GND) U4.55(GND) U4.56(GND) U4.57(GND) U4.58(GND) U4.59(GND) U4.60(GND) U4.61(GND) U4.62(GND) U4.63(GND) U4.64(GND) U4.65(GND) U4.66(GND) U4.67(GND) U4.68(GND) U4.69(GND) U4.70(GND) U4.71(GND) U4.72(GND) U4.73(GND) U4.74(GND) U4.75(GND) U4.76(GND) U4.77(GND) U4.78(GND) U4.79(GND) U4.80(GND) U4.81(GND) U4.82(GND) U4.83(GND) U4.84(GND) U4.85(GND) U4.86(GND) U4.87(GND) U4.88(GND) U4.89(GND) U4.90(GND) U4.91(GND) U4.92(GND) U4.93(GND) U4.94(GND) U4.95(GND) U4.96(GND) U4.97(GND) U4.98(GND) U4.99(GND) U4.100(GND) U4.101(GND) U4.102(GND) U5.10(GND) U5.12(GND) U5.13(GND) U5.24(GND) U8.1(GND) U8.3(GND) U8.5(GND) U8.9(DTR_I) U8.10(RTS_I) U8.14(GND) U8.20(GND) U8.21(GND) U8.22(GND) U8.30(GND) U8.32(GND) U8.43(GND) U8.50(GND) U8.54(GND) U8.55(GND) U8.57(GND) U8.58(GND) U8.60(GND) U8.61(GND) U8.63(GND) U8.64(GND) U8.65(GND) U8.66(GND) U8.67(GND) U8.68(GND) U8.69(GND) U8.70(GND) U8.71(GND) U8.72(GND) U8.73(GND) U8.74(GND) U8.75(GND) U8.76(GND) U8.77(GND) U8.78(GND) U8.79(GND) U8.80(GND) U8.81(GND) U8.82(GND) U8.83(GND) U8.84(GND) U8.85(GND) U8.86(GND) U8.87(GND) U8.88(GND) U8.89(GND) U8.90(GND) U8.91(GND) U8.92(GND) U8.93(GND) U8.94(GND) U8.95(GND) U8.96(GND) U11.2(P$V-) U13.2(P$V-) U14.1(GND) U14.3(GND) U14.4(GND) U14.6(GND) U14.7(GND) U15.11(TEST) U15.EP(GND) U16.7(DIR3) U16.9(!OE) U16.10(GND) U18.3(P$V-) ; also sheet 1
GNSS_!RESET!: C58.1 R64.1 U4.49(!RESET!) U5.8(!RESET!) U18.2(A) ; also sheet 1
LARA_18_NI: U8.16(GPIO1) U16.3(A1)
LARA_18_RXDO: U8.13(RXD_O) U16.4(A2)
LARA_18_TXDI: U8.12(TXD_I) U16.5(A3)
LARA_!RESET!: Q6.3(D) U8.18(RESET_N)
LARA_PWR_ON: Q5.3(D) U8.15(PWR_ON)
N$3: R7.2 U4.40(USB_D+)
N$6: R8.2 U4.39(USB_D-)
N$8: J6.SHLD1(SHLD) J6.SHLD2(SHLD) J6.SHLD3(SHLD) J6.SHLD4(SHLD) SHLD2.2
N$9: R27.1 U4.51(EXTINT)
N$11: R46.1 U4.27(TX2)
N$16: R68.1 U18.4(Y)
N$17: R66.2 U5.6(USB_D+)
N$18: R67.2 U5.5(USB_D-)
N$32: R47.1 U4.26(RX2)
N$33: J6.B5(CC2) R33.2
N$34: J6.A5(CC1) R34.2
N$35: R56.1 U11.1(OUT)
N$36: R6.1 U4.53(TIMEPULSE)
N$38: Q2.5(B) R56.2
N$40: Q2.2(B) R63.2
N$41: R63.1 U13.1(OUT)
N$42: Q6.1(G) R68.2
N$43: I2C1.3 R71.2
N$44: I2C1.1 R72.2
N$46: R9.2 U8.28(USB_D-)
N$47: R10.2 U8.29(USB_D+)
N$48: C63.2 R13.2 U15.33(XTALIN) Y2.3
N$49: C64.2 R13.1 U15.32(XTALOUT) Y2.1
N$50: R12.1 U15.35(RBIAS)
N$51: R14.2 U15.28(SUSP_IND)
N$52: R17.2 U15.25(HS_IND/CFG1)
N$53: C65.1 U15.34(PLLFILT)
N$54: C66.1 U15.14(CRFILT)
N$55: R22.2 U15.30(USBDM_UP)
N$56: R23.2 U15.31(USBDP_UP)
N$61: C82.2 D12.1 LARA_RF1.SIG(SIGNAL)
N$62: C82.1 L2.1 U8.56(ANT)
N$63: C83.2 D13.1 LARA_RF2.SIG(SIGNAL)
N$64: C83.1 L3.1 U8.62(ANT2)
N$65: Q5.1(G) R70.2
NEO_RXI: NEO_RX.1 U5.21(RXD1/PICO)
NEO_TXO: NEO_TX.1 U5.20(TXD1/POCI)
RF: C13.1 D1.1 FB1.2 GNSS_RF.SIG(SIGNAL)
SIM_CLK: C71.1 D11.1 J2.C3(CLK) U8.38(SIM_CLK)
SIM_IO: C74.2 D11.6 J2.C7(I/O) U8.39(SIM_IO)
SIM_RST: C72.2 D11.4 J2.C2(RST) U8.40(SIM_RST)
USB251SCL: R52.2 U15.24(SCL/CFG0) USB251SCL.2
USB251SDA: R44.2 U15.22(SDA) USB251SDA.2
USB_!RESET: C67.1 R18.1 U15.26(!RESET)
V_ANT: C11.1 FB1.1 R55.2 R59.2 R60.2 R61.2 U11.3(+IN) U13.4(-IN) VANT.1
V_USB_2: D8.5(VCC) J6.VBUS1(VBUS) J6.VBUS2(VBUS) R21.2 U8.17(VUSB_DET) VUSB2.1 ; also sheet 1
VBUS_DET: C68.1 R20.2 R21.1 U15.27(VBUS_DET)
VCCIO: C69.1 C70.1 U8.4(V_INT) U16.1(DIR1) U16.2(DIR2) U16.6(A4) U16.8(DIR4) U16.16(VCCA) VCCIO.1
VSIM: C73.1 C75.2 D11.3 J2.C1(VCC) U8.41(VSIM)
ZED_EXTINT: R27.2 R28.1 ZED_EXTINT.1 ; also sheet 1
ZED_RX2: R47.2 RX2.1 ; also sheet 1
ZED_TP: R6.2 TP.1 ; also sheet 1
ZED_TX2: R46.2 TX2.1 ; also sheet 1
Unconnected: D8.4(IO3) D8.6(IO4) J2.C6(VPP) U4.5(ANT_OFF) U4.7(V_RF) U4.19(GEO_STAT) U4.20(RTK_STAT) U4.46(TX_READY) U4.47(D_SEL) U5.2(D_SEL) U5.3(TXD2) U5.4(RXD2) U5.9(VCC_RF) U5.14(ANT_OFF) U5.15(ANT_DETECT) U5.16(!ANT_SHORT!) U5.17(EXT_INT) U8.6(DSR_O) U8.7(RI_O) U8.8(DCD_O) U8.11(CTS_O) U8.19(GPIO6) U8.23(GPIO2) U8.24(GPIO3) U8.25(GPIO4) U8.26(SDA) U8.27(SCL) U8.34(I2S_WA) U8.35(I2S_TXD) U8.36(I2S_CLK) U8.37(I2S_RXD) U8.42(GPIO5) U8.59(ANT_DET) U15.8(USBDM_DN4) U15.9(USBDP_DN4) U15.12(PRTPWR1) U15.13(!OCS1) U15.16(PRTPWR2) U15.17(!OCS2) U15.18(PRTPWR3) U15.19(!OCS3) U15.20(PRTPWR4) U15.21(!OCS4) U16.11(B4)

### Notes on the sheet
- u-blox ZED-F9P | u-blox NEO-D9S | u-blox LARA-R6001
- VCC Range: 3.0 - 3.6V
- VCC Range: 3.0 - 3.6V
- 50Ω
- 50Ω
- 50Ω
- 90Ω | 50Ω
- 90Ω
- 7-bit unshifted I2C address: 0x43
- 7-bit unshifted I2C address: 0x42
- Close jumpers to
  enable pull-ups
- 90Ω
- USB Hub USB-C | USB Hub
- Open Collector
  Outputs
- Open jumper to isolate shield
- SIM
- 7-bit unshifted I²C address: 0x2C
- USB2513, or USB2514 can be used
- Antenna Power
- Antenna Splitter
- 50Ω | 50Ω
- Vcc Max: 5.5V
- 50Ω
- ANT | 50Ω | ANT_ZED
- For non-L-Band products:
  Do Not Populate U14
  Change BYPASS1 & BYPASS2 to PASTE
  (Or solder closed manually)
- Paul Clark
- Vcc Max: 5.5V
- v11

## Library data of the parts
3V3 3V3_SW 3V3_SW2 5V 9% 99% !SAFEBOOT_NEO! !SAFEBOOT_ZED! ANT_DET ANT_SHT DET DTR ETH_CS ETH_INT GND NEO_RX NEO_TX PICO POCI PWREN RTS RX RX2 RXD SCK SCL SCL2 SD_CS SDA SDA2 TP TP_BOOT TP_LED TX TX2 TXD VANT VCCA VCCIO VIN VPOE VUSB VUSB2 ZED_EXTINT ZED_RXI ZED_TXO = SparkFun-Connectors:TEST-POINT: SparkFun Test Points
ACT BOOT_SW LED LINK LOAD RESET_SW SHLD1 SHLD2 = SparkFun-Jumpers:JUMPER-SMT_2_NC_TRACE: Normally closed trace jumper
BOOT RESET = SparkFun-Switches:MOMENTARY-SWITCH-SPST: Momentary Switch (Pushbutton) - SPST; PROD_ID: SWCH-13896
BYPASS1 BYPASS2 = SparkFun-Jumpers:JUMPER-SMT_2_SOIC-PAD_NO-PASTE
C1 C3 C5 C6 C8-C10 C14 C18 C22 C23 C25 C26 C29 C56 C59 C60 = SparkFun-Capacitors:2.2UF: 2.2µF ceramic capacitors; PROD_ID: CAP-07888
C2 C7 C15 C17 C19 C21 C30 C31 C33-C38 C52-C54 C58 C61 C62 C65-C70 C75 C78 = SparkFun-Capacitors:0.1UF: 0.1µF ceramic capacitors; PROD_ID: CAP-08604
C4 C40 C43 = SparkFun-Capacitors:10NF: 0.01uF/10nF/10,000pF ceramic capacitors; PROD_ID: CAP-00867
C11 C13 C71-C74 = SparkFun-Capacitors:47PF: 47pF ceramic capacitors; PROD_ID: CAP-08913
C12 C24 = SparkFun-Capacitors:1.0UF: 1µF ceramic capacitors; PROD_ID: CAP-00868
C16 C48 C57 C76 = SparkFun-Capacitors:100UF-POLAR: 100µF polarized capacitors; PROD_ID: CAP-12547
C20 C32 C39 C55 = SparkFun-Capacitors:10UF: 10.0µF ceramic capacitors; PROD_ID: CAP-11015
C27 C28 = SparkFun-Capacitors:10PF: 10pF ceramic capacitors; PROD_ID: CAP-11812
C41 = SparkFun-Capacitors:4.7UF: 4.7µF ceramic capacitors; PROD_ID: CAP-08280
C42 = SparkFun-Capacitors:1.0NF/1000PF: 1nF/1,000pF ceramic capacitors; PROD_ID: CAP-16238
C44 C45 = SparkFun-Capacitors:6.8NF/6800PF: 5.6nF/5600pF ceramic capacitors; PROD_ID: CAP-16239
C46 = SparkFun-Capacitors:22NF/22,000PF: 0.022uF/22nF/22,000pF ceramic capacitors; PROD_ID: CAP-07885
C47 C49-C51 C77 C84 C85 = SparkFun-Capacitors:10UF: 10.0µF ceramic capacitors; PROD_ID: CAP-14259
C63 C64 = SparkFun-Capacitors:18PF: 18pF ceramic capacitors; PROD_ID: CAP-08267
C79 = SparkFun-Capacitors:15PF: 15pF ceramic capacitors; PROD_ID: CAP-07881
C80 = SparkFun-Capacitors:8.2PF: 8.2pF ceramic capacitors; PROD_ID: CAP-16662
C81 = SparkFun-Capacitors:68PF: 68pF ceramic capacitors; PROD_ID: CAP-14092
C82 C83 = SparkFun-Capacitors:33PF: 33pF ceramic capacitors; PROD_ID: CAP-10142
C86 = SparkFun-Capacitors:47UF-POLAR: 47µF polarized capacitors; PROD_ID: CAP-10547
D1 D3 D12 D13 D15-D20 = SparkFun-DiscreteSemi:PESD0402: ESD protection diode; DIGIKEY_PART: PESD0402-140CT-ND; MOUSE_PART: 650-PESD0402-140; PROD_ID: DIO-15359
D2 = SparkFun-LED:LED-RIGHT-ANGLE-PTH; PROD_ID: DIO-13847
D4-D6 D9 = SparkFun-DiscreteSemi:DIODE-SCHOTTKY: Schottky diode; PROD_ID: DIO-14072
D7 D8 D10 = SparkFun-DiscreteSemi:TVS_DIODE_ARRAY; PROD_ID: IC-13538
D11 = SparkFun-DiscreteSemi:TVS_DIODE_ARRAY_4; PROD_ID: DIO-14095
D14 = SparkFun-DiscreteSemi:DIODE-SCHOTTKY: Schottky diode; PROD_ID: DIO-09886; VALUE: 3A/40V/500mV
ESP32_RF = SparkFun-RF:ANTENNA-SMA-GROUNDED: SMA Antenna Connector w/ Ground; PROD_ID: CONN-00827
F1 = SparkFun-Fuses:PPTC: Resettable Fuse PPTC; PROD_ID: RES-14313
FB1 = SparkFun-Coils:FERRITE_BEAD: Ferrite Bead (blocks, cores, rings, chokes, etc.); PROD_ID: NDUC-14988
FB2 = SparkFun-Coils:FERRITE_BEAD: Ferrite Bead (blocks, cores, rings, chokes, etc.); PROD_ID: NDUC-12579
FD1-FD4 = SparkFun-Aesthetics:FIDUCIAL: Fiducial Alignment Points
FRAME1 FRAME2 = SparkFun-Aesthetics:FRAME-LEDGER: Schematic Frame - Ledger
GNSS_RESET = SparkFun-Jumpers:JUMPER-COMBO_2_NO
GNSS_RF LARA_RF1 LARA_RF2 = SparkFun-RF:ANTENNA-SMA-GROUNDED: SMA Antenna Connector w/ Ground; PROD_ID: CONN-08289
H1-H6 = SparkFun-Hardware:STAND-OFF: Stand Off
I2C I2C1 = SparkFun-Jumpers:JUMPER-SMT_3_NO: Normally open jumper This jumper has three pads in close proximity to each other. Apply solder to close the connection(s).
J1 J6 = SparkFun-Connectors:USB_C: USB Type C 16Pin Connector Super Speed pins not available on the 16-pin purely SMD connector so this part is best for USB 2.0 implementations. D1 and D2 are tied together enabling D+/- no matter which way the cable is plugged into the connector. The two channel configuration pins (CC1/2) are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; PROD_ID: CONN-14122
J2 = SparkFun-Connectors:SIMHOLDER: SIM Cellular Card Socket SMT 6 pin standard connection. SparkFun Products: SIM Socket SparkFun Cellular Shield - MG2639 SparkFun SIM Card Socket Breakout; PROD_ID: CONN-16272
J3 = SparkFun-Connectors:MICRO-SD: microSD Socket for Transflash Various sockets for µSD. tDoc lines correctly indicate media card edge positions when inserting (unlocked, locked, depressed). NOTE: CD1 and CD2 are connected internally, and the default detect state of the socket is detect pin to ground. SparkFun Products: WAV Trigger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; PROD_ID: CONN-16110
J4 = SparkFun-Connectors:QWIIC_CONNECTOR: SparkFun I2C Standard Qwiic Connector An SMD 1mm pitch JST connector makes it easy and quick (get it? Qwiic?) to connect I2C devices to each other. The Qwiic system enables fast and solderless connection between popular platforms and various sensors and actuators. We carry 200mm, 100mm, 50mm, and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; PROD_ID: CONN-14483
J8 = SparkFun-Connectors:U.FL2PIN: SMD Antenna Connector - U.FL; PROD_ID: CONN-09193
J9 = SparkFun-Connectors:MAGJACK-POE: MAGJACK: RJ-45 with POE and LEDs This is a single port, RJ45 ethernet jacks with built in transformer (magnetics), PoE rectifier diodes, status LEDs, and shielding.; PROD_ID: CONN-16253
J13 = SparkFun-Connectors:CONN_10: Multi connection point. Often used as Generic Header-pin footprint for 0.1 inch spaced/style header connections On any of the 0.1 inch spaced packages, you can populate with these: Break Away Headers - Straight (PRT-00116) Break Away Male Headers - Right Angle (PRT-00553) Female Headers (PRT-00115)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; PROD_ID: CONN-17279; STOREFRONT: PRT-21328
L1 L4 = SparkFun-Coils:INDUCTOR: Inductors; PROD_ID: NDUC-14234
L2 L3 = SparkFun-Coils:DNP
LOGO1 = SparkFun-Aesthetics:SPECIAL_INSTRUCTIONS: Special Ordering/Production Instructions Alert
LOGO4 = SparkFun-Aesthetics:OSHW-LOGO: Open-Source Hardware (OSHW) Logo
LOGO5 = SparkFun-Aesthetics:SFE_LOGO_NAME: SparkFun Font Logo
LOGO6 = SparkFun-Aesthetics:SFE_LOGO_FLAME: SparkFun Flame Logo
MEAS PW+ PW- VIN+ VIN- = SparkFun-Jumpers:JUMPER-COMBO_2_NC_TRACE
PM0 PM1 PM2 USB251SCL USB251SDA = SparkFun-Jumpers:JUMPER-SMT_2_NO: Normally open jumper
Q1 Q2 = SparkFun-DiscreteSemi:TRANS_NPN_DUAL: Dual NPN Transistors in Single Package The MBT3904W1 puts two general purpose 3904 NPN transistors in a single package. Datasheet SparkFun Products: SparkFun ESP32 Thing; PROD_ID: TRANS-13337
Q5 Q6 = SparkFun-DiscreteSemi:MOSFET-NCH: N-channel MOSFETs Voltage controlled devices that allow control of high current outputs. SparkFun Products: SparkFun OpenScale SparkFun Digital Sandbox SparkFun Monster Moto Shield SparkFun MOSFET Power Controller; PROD_ID: TRANS-11151
R1 R2 R33 R34 = SparkFun-Resistors:5.1KOHM; PROD_ID: RES-12083
R3-R5 R11 R15 R28 R30-R32 R49 R54 R57 R58 R64 VID1 = SparkFun-Resistors:10KOHM: 10kΩ resistor; PROD_ID: RES-00824
R6 R27 R36-R39 R46 R47 = SparkFun-Resistors:33OHM: 33Ω resistor; PROD_ID: RES-08270
R7-R10 R22 R23 R66 R67 = SparkFun-Resistors:27OHM: 27Ω resistor; PROD_ID: RES-09334
R12 = SparkFun-Resistors:12KOHM: 12kΩ resistor; PROD_ID: RES-10327
R13 R24 = SparkFun-Resistors:1MOHM: 1MΩ resistor; PROD_ID: RES-07868
R14 R17 R18 R20 R21 R44 R48 R50-R52 R65 R69 = SparkFun-Resistors:100KOHM: 100kΩ resistor; PROD_ID: RES-07828
R16 R19 R71 R72 = SparkFun-Resistors:2.2KOHM: 2.2kΩ resistor; PROD_ID: RES-08272
R25 R26 R53 R56 R63 R68 R70 VID2 = SparkFun-Resistors:1KOHM: 1kΩ resistor; PROD_ID: RES-07856
R29 = SparkFun-Resistors:12.4KOHM: 12.4kΩ resistor; PROD_ID: RES-16236
R35 R40-R42 = SparkFun-Resistors:49.9OHM: 49.9Ω resistor; PROD_ID: RES-16237
R43 = SparkFun-Resistors:10OHM: 10Ω resistor; PROD_ID: RES-12581
R45 R55 R59-R61 = SparkFun-Resistors:49.9OHM: 49.9Ω resistor; PROD_ID: RES-16252
R62 = SparkFun-Resistors:470OHM: 470Ω resistor; PROD_ID: RES-07869
SPWR TPWR = SparkFun-Jumpers:JUMPER-SMT_3_1-NC_TRACE: Normally closed trace jumper (1 of 2 connections) This jumper has a trace between two pads so it's normally closed (NC). The other connection is normally open (NO). Use a razor knife to open the connection. For best results follow the IPC guidelines for cutting traces: Cutout at least 0.063 mm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
U1 = SparkFun-RF:ESP32-WROVER-E/IE: ESP32-WROVER-E/IE ESP32-WROVER-E uses the onboard antenna. ESP32-WROVER-IE has a u.FL antenna connector, but is otherwise the same as the -E. N16R8 has 16M Flash, 8M PSRAM; PROD_ID: IC-19265
U2 = SparkFun-IC-Comms:CH340C; PROD_ID: IC-14038
U3 U6 = SparkFun-IC-Power:XC6222; IOUT: 700mA; PROD_ID: VREG-16775; VOUT: 3.3V
U4 = SparkFun-GPS:U-BLOX_ZED-F9P; PROD_ID: IC-14209
U5 = SparkFun-GPS:U-BLOX_NEO-D9S: u-blox NEO-D9S The NEO-D9S can receive the data stream of a GNSS correction service, broadcast via satellite L band and compliant to the specification the product is designed for. Integrated with a high precision GNSS receiver, such as from the u-blox F9 platform, it enables the positioning system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; PROD_ID: IC-16579
U7 = SparkFun-IC-Comms:W5500; PROD_ID: IC-16240
U8 = SparkFun-RF:LARA-R6: u-blox LARA-R6 single or multi-mode LTE Cat 1 modules; PROD_ID: IC-16661
U9 = SparkFun-IC-Logic:74LVC4066D_QUAD_BILATERAL_SWITCH: Nexperia Quad Bilateral Switch The 74LVC4066 is a high-speed Si-gate CMOS device. The 74LVC4066 provides four single pole, single-throw analog switch functions. Each switch has two input/output terminals (nY and nZ) and an active HIGH enable input (nE). When nE is LOW, the analog switch is turned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; PROD_ID: IC-13944
U10 = SparkFun-IC-Power:POE_PSU: A special function Power Over Ethernet module with 5V or 12V output. Comes in an SMD package.; PROD_ID: IC-16251
U11 U13 = SparkFun-IC-Amplifiers:MCP6021: MCP6021T-E/OT OP AMP Rail-to-rail input/output op-amp with 10 MHz bandwidth. SparkFun Products ZX Distance and Gesture Sensor (SEN-12780); PROD_ID: IC-12504
U12 = SparkFun-IC-Power:AP7361C-33FGE: AP7361C 3.3V LDO Regulator; PROD_ID: VREG-14094
U14 = SparkFun-RF:BP2G1+_POWER_SPLITTER: BP2G1+ 2 Ways MMIC DC Pass Power Splitter, 1200 - 2000 MHz, 50Ω; PROD_ID: IC-17198
U15 = SparkFun-IC-Special-Function:USB251XB: USB 2.0 Hi-Speed Hub Controller USB2514B is four-port; PROD_ID: IC-15827
U16 = SparkFun-IC-Comms:SN74AVC4T774PW: Texas Instruments,SN74AVC4T774PW,IC, Texas Instruments SN74AVC4T774PW, Dual, Bus Transceiver, 4-Bit Non-Inverting 3-State, 1.2 3.6 V, 16-Pin TSSOP Source: Datasheet; PROD_ID: IC-15360
U17 = SparkFun-IC-Power:URB_YMD-15WR3: MORNSUN DC/DC Converter URB_YMD-15WR3 URB2405YMD-15WR3: Input 24V (9V-36V), Output 5.0V 3.0A; PROD_ID: COMP-19263
U18 = SparkFun-IC-Logic:74*1G04: Single Inverter IC NOT GATE INVERTER SNGL 1IN SOT353 Supply: 1.65V to 5.5V Datasheet SparkFun Products SparkFun Stepoko (ROB-13899) SparkFun CryptoShield (DEV-13183) SparkFun LogicBlocks Kit (KIT-11006) SparkFun ArduMoto (DEV-09815); PROD_ID: COMP-08268
Y1 = SparkFun-Clocks:CRYSTAL-25MHZ: 25MHz Crystal; PROD_ID: XTAL-16235
Y2 = SparkFun-Clocks:CRYSTAL-24MHZ: 24MHz Crystal; PROD_ID: XTAL-14845

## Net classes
2 3.3V: width 0.508 mm
3 RF_IN: width 0.35 mm, clearance 0.46 mm
4 USB: width 0.203 mm, clearance 0.127 mm
7 V_ZED: width 0.2 mm, clearance 0.2 mm
8 V_RF: width 0.2 mm
11 ZED_DIG: width 0.1 mm, clearance 0.1 mm

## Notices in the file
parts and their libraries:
SparkFun-Aesthetics: Licensing: Creative Commons ShareAlike 4.0 International - https://creativecommons.org/licenses/by-sa/4.0
SparkFun-Aesthetics: Released under the Creative Commons Attribution Share-Alike 4.0 License
SparkFun-Aesthetics: https://creativecommons.org/licenses/by-sa/4.0
